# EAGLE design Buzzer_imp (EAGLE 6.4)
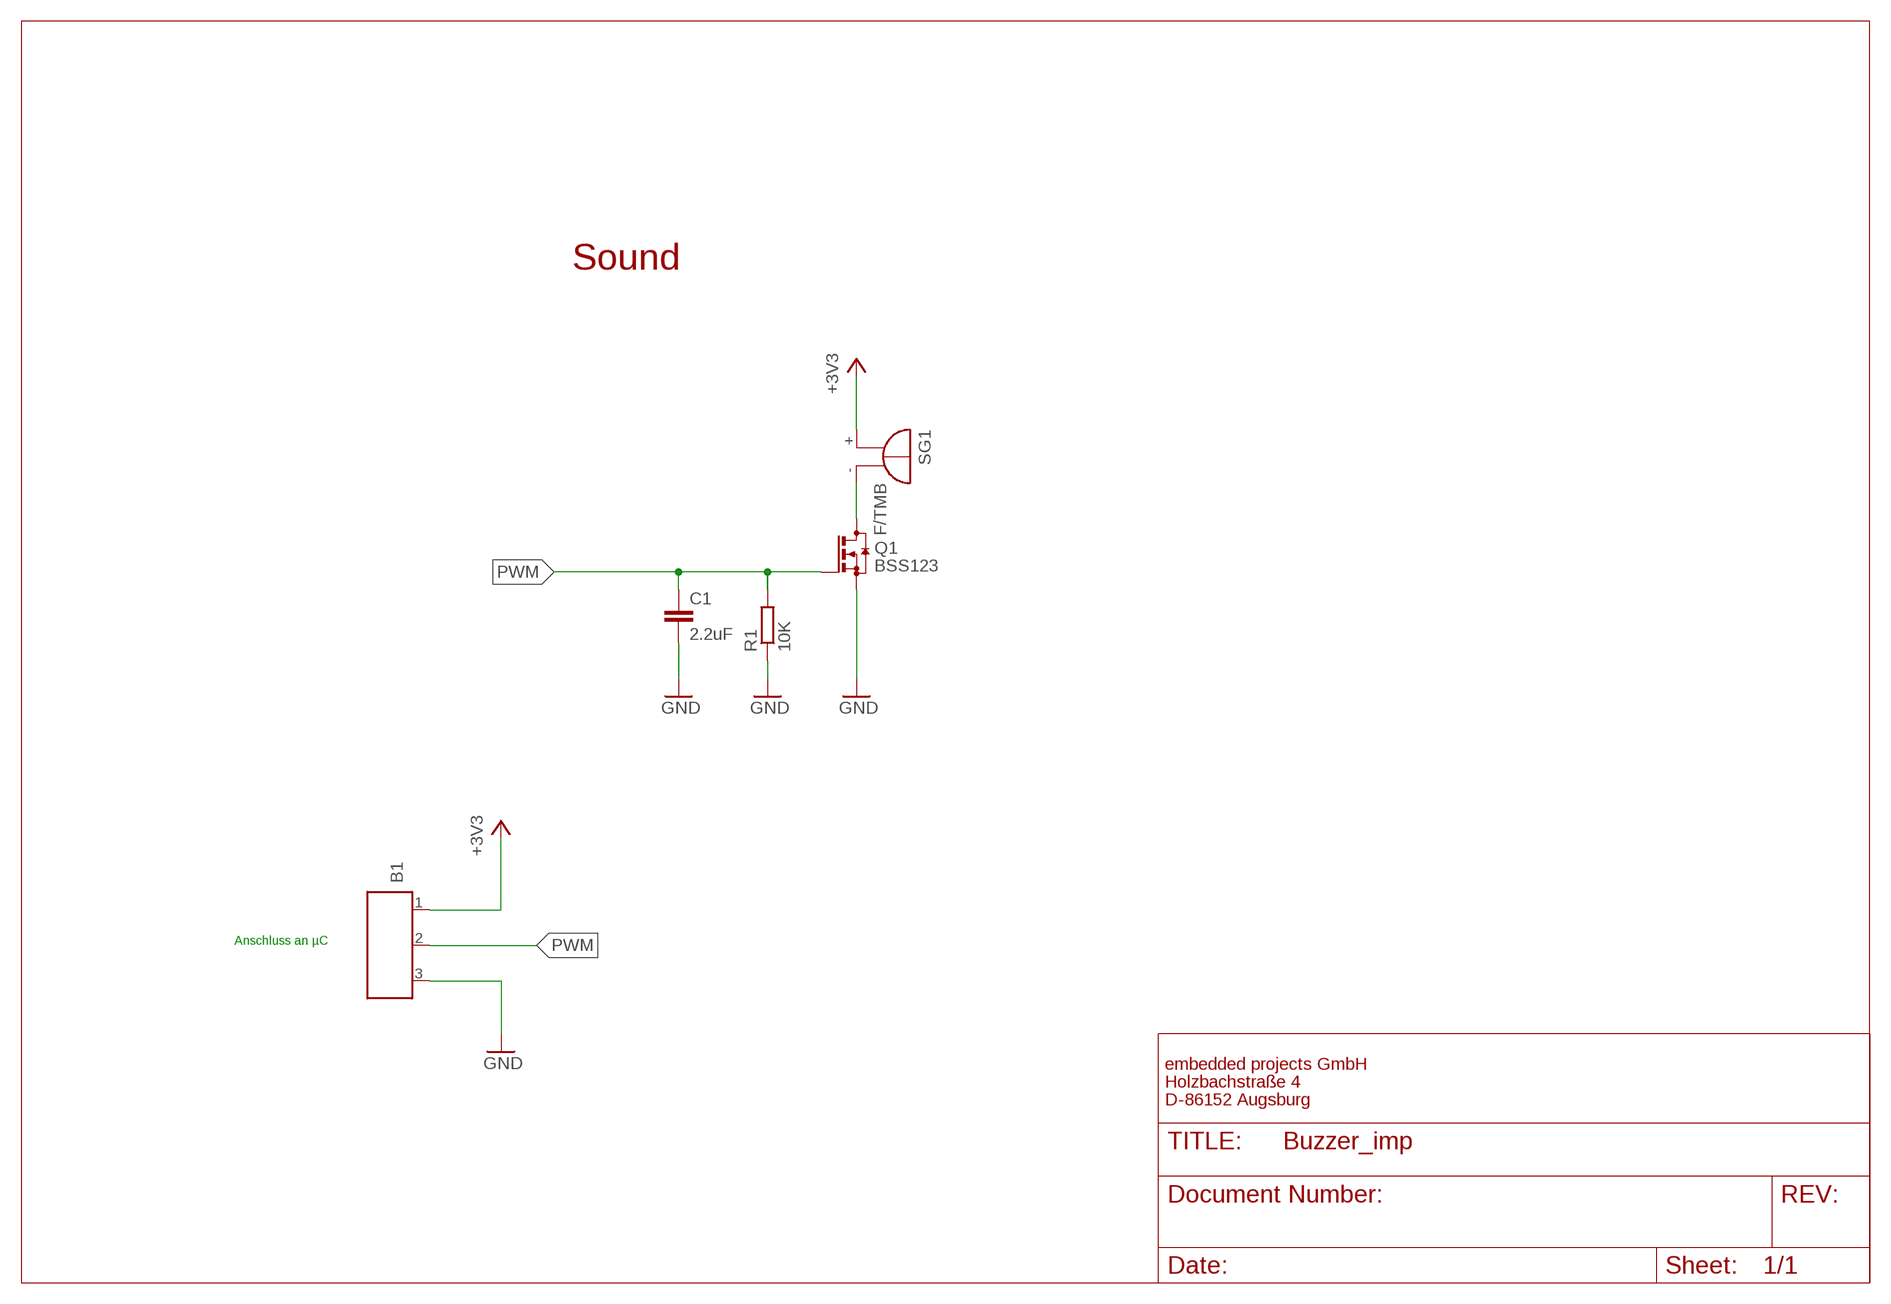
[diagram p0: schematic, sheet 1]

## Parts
B1  MESSFUEHLER_3  [MESSFUEHLER_3]
C1  2.2uF  C-EUC0805  [C0805]
Q1  BSS123  [SOT-23]
R1  10K  R-EU_R0805  [R0805]
SG1  F/TMB  [F/TMB]

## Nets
+3V3: B1.1 SG1.+
GND: B1.3 C1.2 Q1.2(S) R1.1
N$22: Q1.3(D) SG1.-
PWM: B1.2 C1.1 Q1.1(G) R1.2

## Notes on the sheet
- Sound
- Anschluss an µC
- embedded projects GmbH
- Holzbachstraße 4
- D-86152 Augsburg

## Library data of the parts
B1 = e-messfuehler:MESSFUEHLER_3: Messfühler mit drei Anschlüssen, 2 Versorgung, 1 Signal
C1 = rcl:C-EU: CAPACITOR, European symbol
Q1 = EmbeddedProjectsBauteile:BSS123: N-CHANNEL MOS FET; EP: 400196
R1 = rcl:R-EU_: RESISTOR, European symbol
SG1 = buzzer:F/TMB: BUZZER; OC_FARNELL: unknown; OC_NEWARK: unknown

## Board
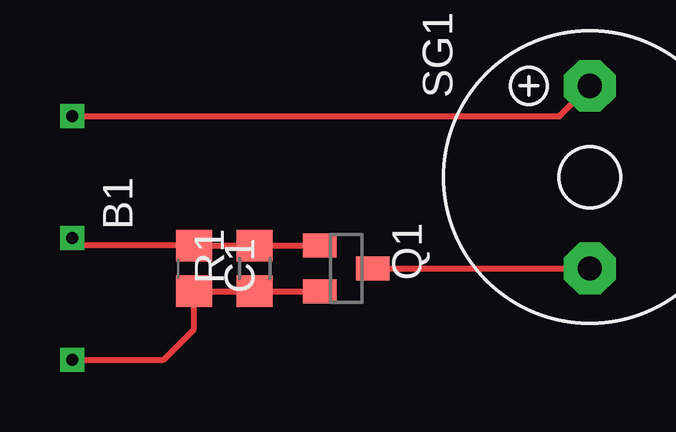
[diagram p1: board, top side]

No outline drawn. Coordinates in mm, seen from the top.
Copper layers (1*16): Top 0.035mm / dielectric 1.5mm / Bottom 0.035mm
Design rules "default": minimum track width 10mil, minimum drill 24mil, track to track 8mil, track to pad 8mil, pad to pad 8mil, via to via 8mil, smd to smd 8mil, copper to edge 40mil, drill to drill 8mil, minimum pad ring 10mil, minimum via ring 8mil, stop-mask expansion 4mil, vias tented up to drill 0mil, thermal gap 10mil

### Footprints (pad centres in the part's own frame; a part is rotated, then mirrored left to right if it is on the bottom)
MESSFUEHLER_3 = drill 0.5 pad 1 square: 1 -5.08,0; 2 0,0; 3 5.08,0
C0805 = smd 1.3 x 1.5: 1 -0.95,0; 2 0.95,0
SOT-23 = smd 1 x 1.4: 1 -0.95,-1.1; 2 0.95,-1.1; 3 0,1.1
R0805 = smd 1.3 x 1.5: 1 -0.95,0; 2 0.95,0
F/TMB = drill 1.016 pad 2.159 octagon: + 3.81,0; - -3.81,0

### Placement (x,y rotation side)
B1  2.54,15.24 270 top
C1  7.62,13.97 270 top
Q1  13.97,13.97 270 top
R1  10.16,13.97 90 top
SG1  24.13,17.78 90 top

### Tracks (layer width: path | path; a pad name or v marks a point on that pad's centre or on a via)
+3V3
  Top 0.254: B1.1 22.86,20.32 SG1.+
GND
  Top 0.254: Q1.2 R1.1 C1.2 7.62,11.43 6.35,10.16 B1.3
N$22
  Top 0.254: Q1.3 SG1.-
PWM
  Top 0.254: Q1.1 R1.2 C1.1 2.86,14.92 B1.2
